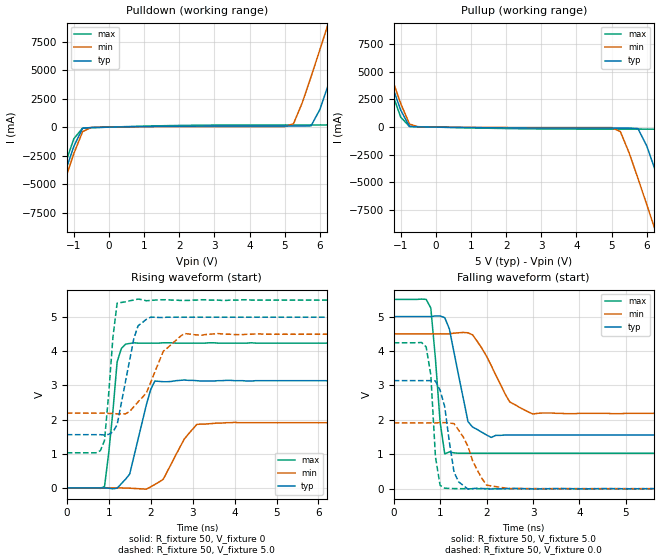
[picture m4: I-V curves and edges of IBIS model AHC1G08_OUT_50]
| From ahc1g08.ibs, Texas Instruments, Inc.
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|   Model AHC1G08_OUT_50
[Model]   AHC1G08_OUT_50
Model_type  Output
Polarity   Inverting
Vmeas = 2.50v
Cref = 15pf
| variable   typ   min   max
C_comp   3.12pf   2.34pf   3.90pf
[Temperature Range]   25   85   -40
[Voltage Range]   5.0   4.5   5.5
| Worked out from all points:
|   slope of the pulldown table from 0 to 0.75 V, typ, clamps not added: 18.8 ohm
|   slope of the pullup table from 0 to 0.75 V, typ, clamps not added: 25.3 ohm
|   rising waveform, R_fixture 50, V_fixture 0: 20-80 % time 371ps typ, 512ps min, 198ps max; typ from 0 V to 3.14 V
|   falling waveform, R_fixture 50, V_fixture 5.0: 20-80 % time 307ps typ, 524ps min, 158ps max; typ from 5 V to 1.56 V
|   rising waveform, R_fixture 50, V_fixture 5.0: 20-80 % time 326ps typ, 537ps min, 181ps max; typ from 1.56 V to 5 V
|   falling waveform, R_fixture 50, V_fixture 0.0: 20-80 % time 211ps typ, 380ps min, 119ps max; typ from 3.14 V to 0 V
[Pulldown]
|   Voltage   I(typ)   I(min)   I(max)
-5V       -40.9A     -41.4A     -40.3A
-1.75V    -8.76A     -9.39A     -8.09A
-1V       -1.69A     -2.33A     -1.02A
-750mV    -95.5mA    -395mA     -80.6mA
5.25V     93.4mA     298mA      192mA
5.75V     116mA      4.42A      192mA
6.25V     3.8A       9.19A      193mA
6.5V      6.17A      11.6A      931mA
6.75V     8.59A      14.1A      3.15A
7.25V     13.5A      19A        7.96A
7.5V      15.9A      21.4A      10.4A
10V       40.7A      46.2A      35.2A
[Pullup]
|   Voltage   I(typ)   I(min)   I(max)
-5V       40.7A      41.2A      40.1A
-2V       11A        11.6A      10.4A
-1.75V    8.59A      9.19A      7.96A
-1V       1.54A      2.14A      907mA
-750mV    63.6mA     284mA      62.5mA
5.25V     -84.4mA    -401mA     -178mA
5.75V     -130mA     -4.62A     -178mA
6.25V     -3.97A     -9.39A     -187mA
6.75V     -8.76A     -14.3A     -3.28A
7.25V     -13.6A     -19.2A     -8.09A
7.5V      -16.1A     -21.6A     -10.5A
10V       -40.9A     -46.4A     -35.3A
[Ramp]
| variable   typ   min   max
dV/dt_r   1.88E+00/3.25E-10   1.15E+00/5.04E-10   2.55E+00/2.32E-10
dV/dt_f   2.09E+00/3.49E-10   1.42E+00/5.52E-10   2.70E+00/1.34E-10
R_load = 50
[Rising Waveform]
R_fixture = 50
V_fixture = 0
|   Time   V(typ)   V(min)   V(max)
0s        0V         0V         0V
900ps     921uV      356uV      40.9mV
1ns       -7.91mV    713uV      1.03V
1.2ns     -5.49mV    1.67mV     3.69V
1.3ns     124mV      -387uV     4.08V
1.5ns     407mV      -7.27mV    4.23V
1.6ns     918mV      -14.4mV    4.25V
2.1ns     3.13V      103mV      4.24V
3.2ns     3.13V      1.87V      4.24V
25ns      3.14V      1.91V      4.24V
[Falling Waveform]
R_fixture = 50
V_fixture = 5.0
V_fixture_min = 4.5
V_fixture_max = 5.5
|   Time   V(typ)   V(min)   V(max)
0s        5V         4.5V       5.5V
800ps     5V         4.5V       5.25V
1ns       5.02V      4.5V       1.94V
1.1ns     4.97V      4.5V       1.01V
1.2ns     4.64V      4.5V       1.07V
1.6ns     1.95V      4.53V      1.03V
2.1ns     1.49V      3.58V      1.03V
2.5ns     1.56V      2.52V      1.03V
3ns       1.56V      2.17V      1.03V
25ns      1.56V      2.19V      1.03V
[Rising Waveform]
R_fixture = 50
V_fixture = 5.0
V_fixture_min = 4.5
V_fixture_max = 5.5
|   Time   V(typ)   V(min)   V(max)
0s        1.56V      2.19V      1.03V
800ps     1.56V      2.19V      1.09V
900ps     1.55V      2.19V      1.39V
1.1ns     1.64V      2.18V      4.41V
1.2ns     1.85V      2.17V      5.41V
1.7ns     4.75V      2.52V      5.53V
1.9ns     4.94V      2.79V      5.48V
2.3ns     4.99V      4V         5.51V
2.8ns     5V         4.52V      5.49V
25ns      5V         4.5V       5.5V
[Falling Waveform]
R_fixture = 50
V_fixture = 0.0
|   Time   V(typ)   V(min)   V(max)
0s        3.14V      1.91V      4.24V
700ps     3.14V      1.91V      4.12V
800ps     3.14V      1.91V      3.31V
900ps     3.13V      1.91V      925mV
1.1ns     2.38V      1.92V      13.8mV
1.3ns     482mV      1.89V      3.07mV
1.6ns     -13.6mV    1.23V      -2.05mV
2ns       -4.59mV    103mV      1.17mV
2.5ns     6.84mV     3.35mV     -994uV
25ns      0V         0V         0V
